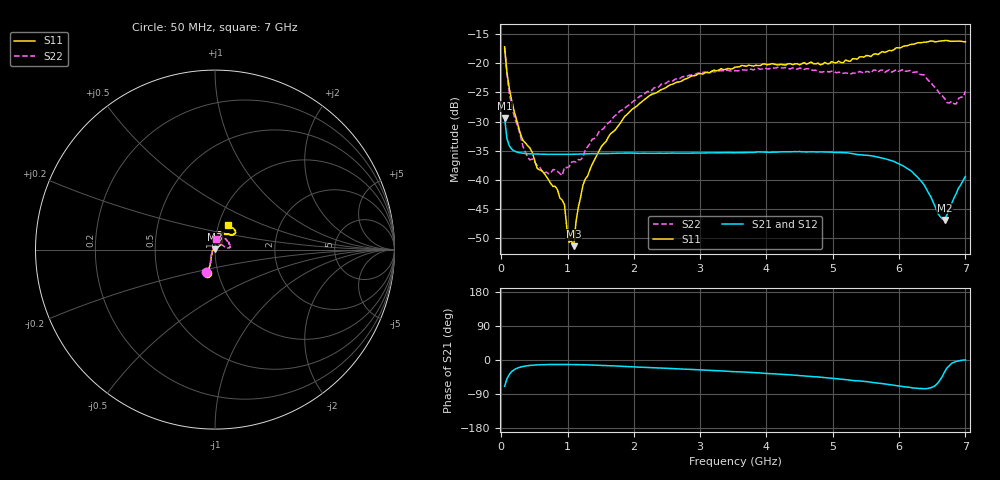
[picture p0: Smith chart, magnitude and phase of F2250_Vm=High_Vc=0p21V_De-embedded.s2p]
! Integrated Device Technology
! Corporate Headquarters
! 6024 Silver Creek Valley Road
! San Jose, CA 95138  USA
! Phone:  1-408-284-8200
! Toll Free:  1-800-223-1366
! Webpage:  http://www.idt.com/
! Timing and RF Division
! 515 Groton Road, Suite 102
! Westford, MA 01886-6024
! Device:  F2250
! Description: Voltage Variable RF Attenuator
! Frequency:  50.0 -  6000.00 MHz
! Package:  3x3 mm Thin QFN Plastic Package: 16 pin
! Ports:  2 RF, 3 DC
!  Pin  1  = GND
!  Pin  2  = NC
!  Pin  3  = RF1  = Port 1
!  Pin  4  = NC
!  Pin  5  = GND
!  Pin  6  = GND
!  Pin  7  = GND
!  Pin  8  = GND
!  Pin  9  = NC
!  Pin 10  = RF2  = Port 2
!  Pin 11  = NC
!  Pin 12  = GND
!  Pin 13  = GND
!  Pin 14  = VCNTRL
!  Pin 15  = VDD
!  Pin 16  = VMODE
! Vcntrl:  0.210 Volts
! Vmode:  +3.300 Volts
! Vdd:  +3.30  Volts
! Current:  1.244 mA
! Data:  The device was measured on a the F2250 evaluation board which has
!  individual transmission lines to the RF pins.  Data was collected
!  using a calibrated network analyzer.  The evaluation board was
!  de-embedded using a TRL calibration technique.
!  The reference plane is the edge of the package pin.
! Misc:  SN 10
!  Action Tracker AT0258
! Date Measured:  2014-11-26
! Date:  2015-10-15  MJV
! Note:
!  Integrated Device Technology supplies this data as a sample of measured
!  data at the package pin for this product.  Your particular data for this
!  product may vary.
!  Data was taken at 25 degrees C.
!  Integrated Device Technology reserves the right to change this data at anytime.
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# GHz S dB R 50
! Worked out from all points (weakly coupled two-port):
!   201 points, 50 MHz to 7 GHz, reference 50 ohm
!   highest |S21| = -29.38 dB at 50 MHz (marker M1); lowest = -46.8 dB at 6.687 GHz (marker M2)
!   lowest |S11| = -51.3 dB at 1.093 GHz (marker M3), VSWR 1.01, Z = 50 + j0.272 ohm
!   |S11| at or under -10 dB: start of sweep to end of sweep
!   |S22| runs from -39.2 to -17.4 dB; largest |S21 - S12| = 5.3e-05
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0.05  -17.18 -108.5  -29.38 -69.5  -29.38 -69.5  -17.37 -110.6
0.08475  -21.47 -107.4  -32.86 -50.1  -32.86 -50.1  -21.87 -109.1
0.15425  -26.23 -116.6  -34.68 -31.0  -34.68 -31.0  -27.10 -120.7
0.29325  -32.27 -127.4  -35.35 -18.5  -35.35 -18.5  -32.66 -133.5
0.3975  -34.11 -142.2  -35.48 -15.0  -35.47 -15.1  -36.07 -158.4
0.5365  -37.89 -154.7  -35.55 -12.9  -35.55 -12.9  -37.48 -179.9
0.64075  -38.77 -162.5  -35.58 -12.2  -35.58 -12.2  -38.87 160.8
0.91875  -43.43 156.0  -35.60 -11.8  -35.60 -11.8  -39.21 127.9
0.9535  -44.24 170.8  -35.59 -11.8  -35.60 -11.8  -37.81 124.2
1.023  -50.65 140.2  -35.59 -11.9  -35.59 -11.9  -37.72 108.1
1.0925  -51.32 89.3  -35.57 -12.0  -35.58 -12.0  -36.83 98.7
1.12725  -47.10 61.8  -35.56 -12.1  -35.56 -12.1  -36.90 91.7
1.2315  -40.86 41.0  -35.53 -12.5  -35.52 -12.5  -36.05 77.3
1.6485  -32.03 41.2  -35.44 -15.2  -35.44 -15.2  -29.92 60.0
2.37825  -24.75 46.7  -35.40 -21.0  -35.40 -21.0  -24.03 53.9
3.525  -20.65 71.7  -35.31 -30.6  -35.32 -30.6  -21.26 73.0
4.7065  -20.06 72.0  -35.15 -43.9  -35.16 -43.9  -21.21 70.3
5.85325  -17.79 40.5  -36.58 -64.9  -36.58 -64.9  -21.13 23.4
6.27025  -16.52 39.4  -39.40 -74.5  -39.40 -74.6  -21.46 8.6
6.68725  -16.11 47.9  -46.81 -31.0  -46.78 -30.9  -26.03 28.5
6.861  -16.22 54.5  -42.31 -3.7  -42.28 -3.8  -26.96 57.4
7  -16.32 62.4  -39.35 -0.1  -39.32 -0.2  -24.81 83.6
